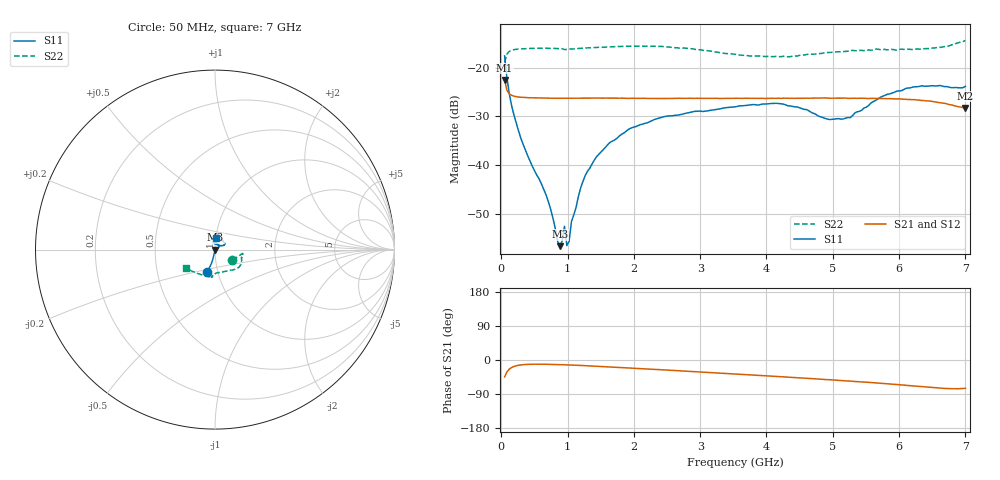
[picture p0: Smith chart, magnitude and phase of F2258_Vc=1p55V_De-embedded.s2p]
! Integrated Device Technology
! Corporate Headquarters
! 6024 Silver Creek Valley Road
! San Jose, CA 95138  USA
! Phone:  1-408-284-8200
! Toll Free:  1-800-223-1366
! Webpage:  http://www.idt.com/
! Timing and RF Division
! 515 Groton Road, Suite 102
! Westford, MA 01886-6024
! Device:  F2258
! Description: Voltage Variable RF Attenuator
! Frequency:  50.0 -  6000.00 MHz
! Package:  3x3 mm Thin QFN Plastic Package: 16 pin
! Ports:  2 RF, 2 DC
!  Pin  1  = NC
!  Pin  2  = NC
!  Pin  3  = RF2  = Port 2
!  Pin  4  = GND
!  Pin  5  = Vdd
!  Pin  6  = NC
!  Pin  7  = VCTRL
!  Pin  8  = NC
!  Pin  9  = GND
!  Pin 10  = RF1  = Port 1
!  Pin 11  = NC
!  Pin 12  = NC
!  Pin 13  = NC
!  Pin 14  = NC
!  Pin 15  = NC
!  Pin 16  = NC
! Vcntrl:  1.550 Volts
! Vdd:  +3.300 Volts
! Current:  1.164 mA
! Data:  The device was measured on a the F2258 evaluation board which has
!  individual transmission lines to the RF pins.  Data was collected
!  using a calibrated network analyzer.  The evaluation board was
!  de-embedded using a TRL calibration technique.
!  The reference plane is the edge of the package pin.
! Misc:  SN 10
!  Action Tracker AT0285
! Date Measured:  2014-12-10
! Date:  2016-01-13  MJV
! Note:
!  Integrated Device Technology supplies this data as a sample of measured
!  data at the package pin for this product.  Your particular data for this
!  product may vary.
!  Data was taken at 25 degrees C.
!  Integrated Device Technology reserves the right to change this data at anytime.
!Freq_(GHz)  S11M_(dB)  S11P_(deg)  S21M_(dB)  S21P_(deg)  S12M_(dB)  S12P_(deg)  S22M_(dB)  S22P_(deg)
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# GHz S dB R 50
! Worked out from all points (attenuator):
!   201 points, 50 MHz to 7 GHz, reference 50 ohm
!   highest |S21| = -22.53 dB at 50 MHz (marker M1); lowest = -28.3 dB at 7 GHz (marker M2)
!   lowest |S11| = -56.6 dB at 884 MHz (marker M3), VSWR 1.00, Z = 50.1 - j0.0439 ohm
!   |S11| at or under -10 dB: start of sweep to end of sweep
!   |S22| runs from -18.9 to -14.4 dB; largest |S21 - S12| = 0.00056
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0.05  -17.58 -108.9  -22.53 -44.7  -22.53 -44.7  -18.92 -30.9
0.1195  -25.22 -102.6  -25.35 -24.2  -25.34 -24.2  -16.66 -10.7
0.2585  -32.91 -102.1  -26.03 -14.0  -26.04 -14.0  -16.17 -7.7
0.6755  -46.13 -88.2  -26.26 -11.3  -26.26 -11.3  -16.00 -12.0
0.884  -56.64 -17.3  -26.27 -12.3  -26.28 -12.3  -16.09 -15.6
0.91875  -55.53 7.1  -26.25 -12.5  -26.27 -12.5  -16.10 -16.3
0.9535  -52.55 -94.5  -26.27 -12.6  -26.26 -12.7  -16.28 -16.2
0.98825  -56.51 -84.5  -26.27 -12.9  -26.25 -12.9  -16.26 -17.0
1.023  -55.65 -32.9  -26.29 -13.1  -26.27 -13.1  -16.19 -17.6
1.05775  -51.60 -13.8  -26.28 -13.3  -26.29 -13.3  -16.15 -18.0
1.2315  -43.36 14.6  -26.25 -14.6  -26.25 -14.6  -15.99 -20.7
1.44  -38.23 17.6  -26.23 -16.7  -26.26 -16.7  -15.86 -23.8
1.6485  -35.26 21.4  -26.26 -18.6  -26.27 -18.6  -15.73 -26.7
2.37825  -30.33 41.0  -26.32 -25.3  -26.32 -25.3  -15.64 -36.9
3.525  -28.04 88.3  -26.29 -36.8  -26.36 -36.7  -17.28 -61.0
4.1505  -27.32 103.6  -26.30 -43.4  -26.35 -43.3  -17.67 -80.2
4.7065  -29.34 93.9  -26.22 -49.3  -26.26 -49.3  -17.24 -91.8
4.94975  -30.64 77.0  -26.27 -52.0  -26.32 -51.9  -16.88 -93.9
5.2625  -30.26 49.3  -26.30 -55.6  -26.32 -55.5  -16.51 -96.0
5.85325  -25.39 26.5  -26.36 -63.3  -26.41 -63.3  -16.33 -98.7
6.33975  -23.72 32.6  -26.73 -70.5  -26.79 -70.5  -16.20 -109.6
7  -23.83 83.6  -28.27 -74.7  -28.37 -74.7  -14.41 -147.3
